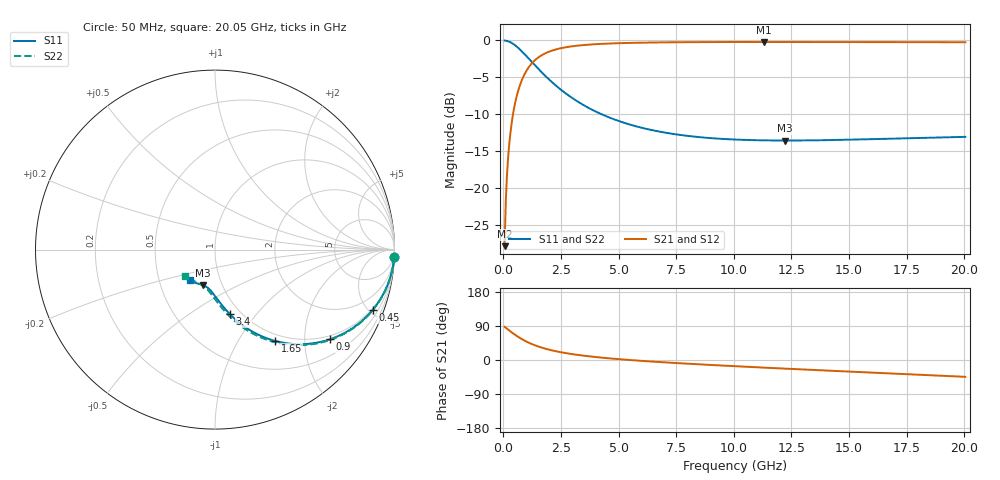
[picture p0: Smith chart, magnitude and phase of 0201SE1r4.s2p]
! AVX Thin Film Operation		Date: August 2001
! Description: Accu-P® Series, Thin Film, SMD, RF Capacitor
! Part Number: 02013J1R4ABW
! 50 MHz  -  20.05 GHz
! Serial Measurements
# mhz S db R 50
!	S11		S21		S12		S22
!	dB	Phase	dB	Phase	dB	Phase	dB	Phase
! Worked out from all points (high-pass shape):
!   401 points, 50 MHz to 20.05 GHz, reference 50 ohm
!   highest |S21| = -0.21 dB at 11.3 GHz (marker M1); lowest = -27.9 dB at 50 MHz (marker M2)
!   |S21| within 3 dB of the highest: 1.204 GHz to end of sweep
!   lowest |S11| = -13.6 dB at 12.2 GHz (marker M3), VSWR 1.53, Z = 40.5 - j16.7 ohm
!   |S11| at or under -10 dB: 4.244 GHz to end of sweep
!   |S22| runs from -13.6 to 0.0 dB; largest |S21 - S12| = 0
!   S11 on the Smith chart (normalised r, x): 50 MHz: 1, -47; 450 MHz: 0.90, -5.24; 900 MHz: 0.90, -2.63; 1.65 GHz: 0.90, -1.45; 3.4 GHz: 0.89, -0.74; 20.05 GHz: 0.72, -0.26
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50  -0.01 -2.4  -27.93 87.6  -27.93 87.6  -0.01 -2.5
100  -0.03 -4.9  -21.93 85.1  -21.93 85.1  -0.03 -4.9
200  -0.11 -9.6  -15.99 80.3  -15.99 80.3  -0.11 -9.8
250  -0.17 -12.0  -14.12 77.9  -14.12 77.9  -0.17 -12.1
350  -0.33 -16.6  -11.36 73.3  -11.36 73.3  -0.33 -16.8
450  -0.53 -21.0  -9.38 68.8  -9.38 68.8  -0.53 -21.3
650  -1.04 -29.2  -6.71 60.6  -6.71 60.6  -1.04 -29.5
900  -1.81 -38.0  -4.68 51.7  -4.68 51.7  -1.81 -38.5
1200  -2.81 -46.7  -3.23 42.9  -3.23 42.9  -2.81 -47.4
1650  -4.30 -56.6  -2.03 32.8  -2.03 32.8  -4.30 -57.5
2000  -5.36 -62.4  -1.50 26.9  -1.50 26.9  -5.36 -63.5
2400  -6.45 -67.7  -1.13 21.6  -1.13 21.6  -6.45 -69.0
2850  -7.53 -72.4  -0.86 16.7  -0.86 16.7  -7.53 -73.9
3400  -8.64 -76.9  -0.65 12.0  -0.65 12.0  -8.64 -78.7
4950  -10.88 -86.0  -0.38 2.5  -0.38 2.5  -10.89 -88.6
6750  -12.37 -93.2  -0.27 -5.3  -0.27 -5.3  -12.38 -96.7
10050  -13.46 -103.4  -0.22 -16.4  -0.22 -16.4  -13.48 -108.4
11300  -13.57 -106.8  -0.21 -20.1  -0.21 -20.1  -13.60 -112.3
12200  -13.59 -109.2  -0.21 -22.7  -0.21 -22.7  -13.62 -115.1
13400  -13.57 -112.3  -0.21 -26.1  -0.21 -26.1  -13.61 -118.8
16750  -13.34 -120.8  -0.23 -35.4  -0.23 -35.4  -13.40 -128.7
20050  -13.09 -129.1  -0.25 -44.4  -0.25 -44.4  -13.16 -138.4
